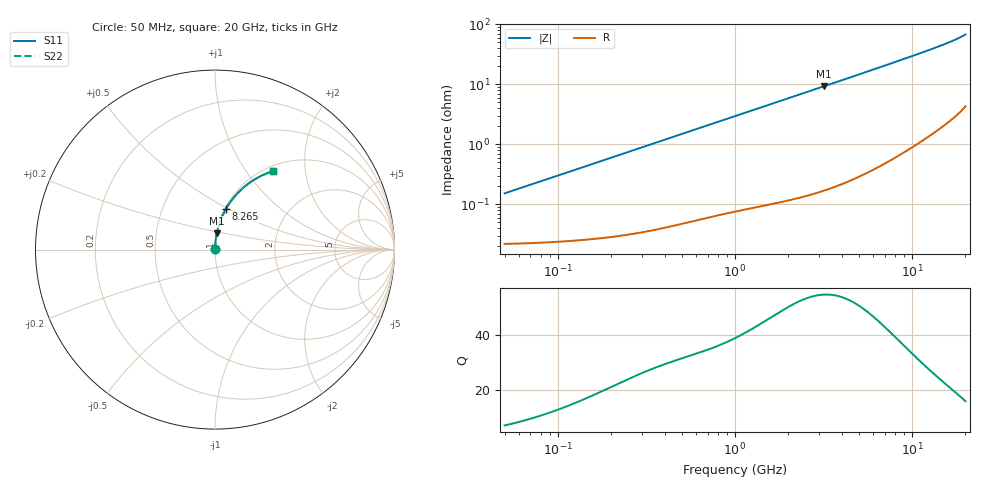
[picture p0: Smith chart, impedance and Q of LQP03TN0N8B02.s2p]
!Murata Part Number: LQP03TN0N8B02
!These Parameters are Measured in Series Mode Connection
!  o--[Z]--o
!Port1  Port2
!  o-------o
!Freq. Start=50[MHz] Stop=20[GHz], 401[Steps]
# Hz S RI R 50
!Freq.(Hz) S11(Real) S11(Imag) S21(Real) S21(Imag) S12(Real) S12(Imag) S22(Real) S22(Imag)
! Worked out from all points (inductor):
!   401 points, 50 MHz to 20 GHz, reference 50 ohm
!   read as one part in series: L = 478 pH near 51.52 MHz
!   highest Q = 54.8 at 3.169 GHz (marker M1), where L = 462 pH
!   S11 on the Smith chart (normalised r, x): 50 MHz: 1.00, +0.00; 8.265 GHz: 1.01, +0.48; 20 GHz: 1.09, +1.35
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5e7  0.00022 0.0015  0.9998 -0.0015  0.9998 -0.0015  0.00022 0.0015
5.152053e7  0.000221 0.00155  0.9998 -0.00155  0.9998 -0.00155  0.000221 0.00155
1.364002e8  0.000269 0.00408  0.9997 -0.00408  0.9997 -0.00408  0.000269 0.00408
3.721004e8  0.000508 0.011  0.9995 -0.011  0.9995 -0.011  0.000508 0.011
1e9  0.00161 0.0292  0.9984 -0.0292  0.9984 -0.0292  0.00161 0.0292
1.714689e9  0.00352 0.0496  0.9965 -0.0496  0.9965 -0.0496  0.00352 0.0496
2.728004e9  0.00766 0.0784  0.9923 -0.0784  0.9923 -0.0784  0.00766 0.0784
3.168813e9  0.01 0.0908  0.99 -0.0908  0.99 -0.0908  0.01 0.0908
3.967106e9  0.0151 0.1131  0.9849 -0.1131  0.9849 -0.1131  0.0151 0.1131
4.966507e9  0.023 0.1405  0.977 -0.1405  0.977 -0.1405  0.023 0.1405
6.125241e9  0.0343 0.1714  0.9657 -0.1714  0.9657 -0.1714  0.0343 0.1714
7.442007e9  0.0496 0.2053  0.9504 -0.2053  0.9504 -0.2053  0.0496 0.2053
8.264682e9  0.0604 0.2256  0.9396 -0.2256  0.9396 -0.2256  0.0604 0.2256
9.457416e9  0.0779 0.254  0.9221 -0.254  0.9221 -0.254  0.0779 0.254
1.082228e10  0.1002 0.2846  0.8998 -0.2846  0.8998 -0.2846  0.1002 0.2846
1.220001e10  0.1251 0.3134  0.8749 -0.3134  0.8749 -0.3134  0.1251 0.3134
1.375312e10  0.156 0.3433  0.844 -0.3433  0.844 -0.3433  0.156 0.3433
1.527346e10  0.1892 0.3699  0.8108 -0.3699  0.8108 -0.3699  0.1892 0.3699
1.670968e10  0.2237 0.3928  0.7763 -0.3928  0.7763 -0.3928  0.2237 0.3928
1.800918e10  0.2586 0.4116  0.7414 -0.4116  0.7414 -0.4116  0.2586 0.4116
1.940974e10  0.3022 0.43  0.6978 -0.43  0.6978 -0.43  0.3022 0.43
2e10  0.3235 0.4371  0.6765 -0.4371  0.6765 -0.4371  0.3235 0.4371
